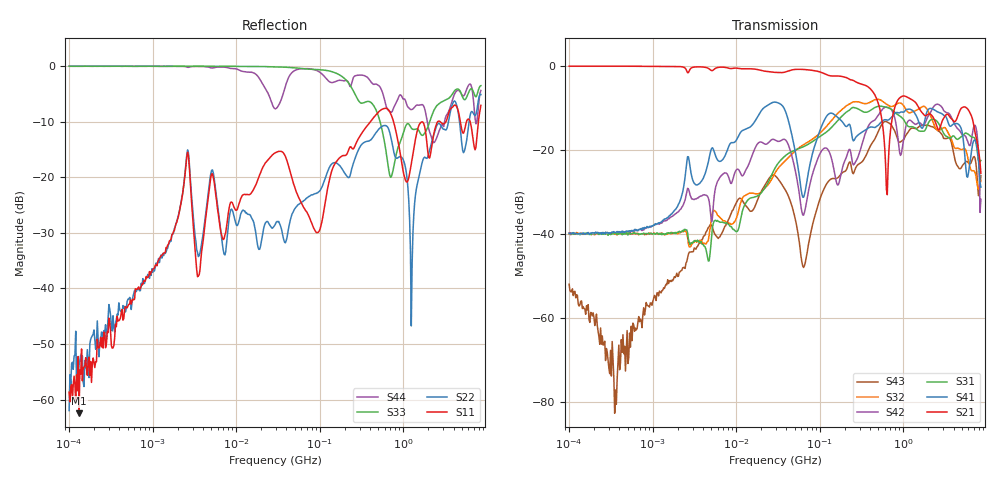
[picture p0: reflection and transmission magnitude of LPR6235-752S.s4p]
# MHz S MA R 50
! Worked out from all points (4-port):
!   498 points, 100 kHz to 8.5 GHz, reference 50 ohm
!   strongest paths, dB at 100 kHz, 1.698 MHz, 29.49 MHz, 500.7 MHz, 8.5 GHz:
!     S21: -0.1, -0.1, -1.5, -8.8, -25.6
!     S41: -39.9, -35.3, -8.6, -14.1, -28.9
!     S31: -40.0, -39.8, -24.2, -9.6, -22.5
!     S42: -39.8, -35.9, -17.7, -11.8, -31.8
!     S32: -40.0, -40.0, -25.3, -7.9, -27.3
!     S43: -52.0, -51.0, -26.2, -15.7, -26.2
!   lowest |S11| = -62.4 dB at 131.5 kHz (marker M1), VSWR 1.00, Z = 50.1 + j0.0337 ohm
!   |S11| at or under -10 dB: 764.5 MHz to 2.592 GHz (1.827 GHz wide, 109 % of centre); 4.819 GHz to 5.727 GHz (908.2 MHz wide, 17.2 % of centre); 6.325 GHz to 7.946 GHz (1.622 GHz wide, 22.7 % of centre)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
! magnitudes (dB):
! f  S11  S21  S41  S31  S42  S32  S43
! 100 kHz  -58.6  -0.1  -39.9  -40.0  -39.8  -40.0  -52.0
! 131.5 kHz  -62.4  -0.1  -40.0  -40.0  -39.9  -39.9  -57.2
! 359.3 kHz  -46.4  0.0  -39.7  -39.8  -39.9  -39.9  -77.2
! 2.62 MHz  -15.5  -1.6  -21.6  -39.7  -29.1  -40.8  -45.8
! 614.9 MHz  -7.6  -23.5  -12.8  -9.8  -9.8  -9.0  -13.2
! 1.248 GHz  -17.6  -8.0  -10.4  -14.5  -13.1  -11.0  -14.9
! 8.5 GHz  -7.1  -25.6  -28.9  -22.5  -31.8  -27.3  -26.2
